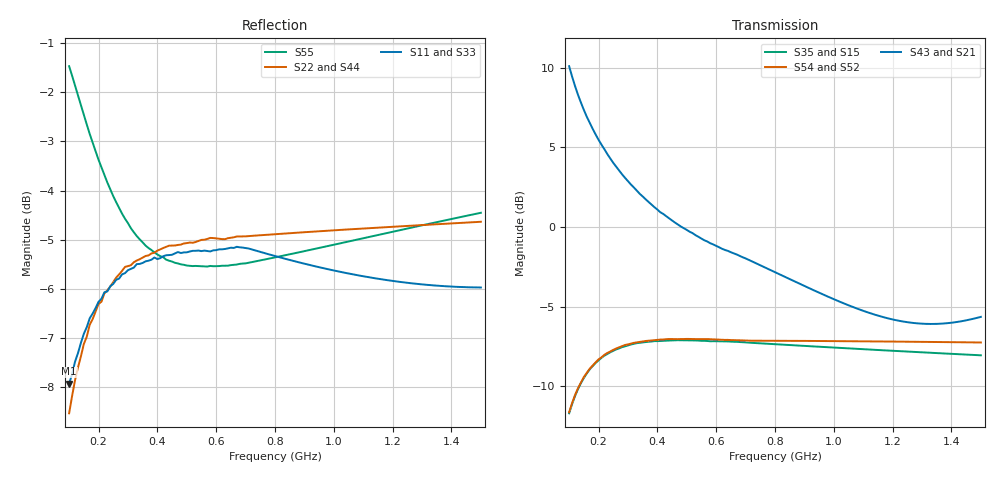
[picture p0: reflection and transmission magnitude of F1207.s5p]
!  POLYFET RF DEVICES
!  S PARAMETER FOR
!  F1207
!  VDS=12.5V IDS=400MA
!  APR 12TH  1996
!AWR Design Environment (2053) Wed Feb 04 14:39:53 2004
!freq-unit  param-type  data-format  keyword  impedance-ohms
# MHz  S  MA  R  50
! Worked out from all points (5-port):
!   141 points, 100 MHz to 1.5 GHz, reference 50 ohm
!   strongest paths, dB at 100 MHz, 450 MHz, 800 MHz, 1.15 GHz, 1.5 GHz:
!     S43: 10.1, 0.4, -2.8, -5.6, -5.6
!     S21: 10.1, 0.4, -2.8, -5.6, -5.6
!     S54: -11.6, -7.0, -7.1, -7.2, -7.3
!     S52: -11.6, -7.0, -7.1, -7.2, -7.3
!     S35: -11.7, -7.1, -7.4, -7.7, -8.1
!     S15: -11.7, -7.1, -7.4, -7.7, -8.1
!   lowest |S11| = -7.9 dB at 100 MHz (marker M1), VSWR 2.34, Z = 31.7 - j29.7 ohm
!   |S11| at or under -10 dB: nowhere
